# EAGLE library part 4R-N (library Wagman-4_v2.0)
Array Chip Resistor Source: RS Component / Phycomp
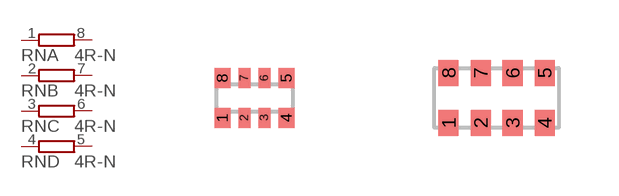
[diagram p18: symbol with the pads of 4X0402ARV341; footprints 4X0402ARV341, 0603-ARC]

Designator prefix RN; gates A=R1NV B=R1NV C=R1NV D=R1NV

## 4R-N0402ARV341 (OC_FARNELL: unknown; OC_NEWARK: unknown)  [4X0402ARV341]
1  A:1  pas
2  B:1  pas
3  C:1  pas
4  D:1  pas
5  D:2  pas
6  C:2  pas
7  B:2  pas
8  A:2  pas

## 4R-N0603-ARC (OC_FARNELL: unknown; OC_NEWARK: unknown)  [0603-ARC]
Pads as for 4X0402ARV341

## 4R-N0603-ARV (OC_FARNELL: unknown; OC_NEWARK: unknown)  [0603-ARV]
Pads as for 4X0402ARV341

## 4R-NCAT16 (OC_FARNELL: unknown; OC_NEWARK: unknown)  [CAT16]
Pads as for 4X0402ARV341

## 4R-NCAY16 (OC_FARNELL: unknown; OC_NEWARK: unknown)  [CAY16]
Pads as for 4X0402ARV341

## 4R-NEXB18V (OC_FARNELL: unknown; OC_NEWARK: unknown)  [EXB18V]
Pads as for 4X0402ARV341

## 4R-NEXB28V (OC_FARNELL: unknown; OC_NEWARK: unknown)  [EXB28V]
Pads as for 4X0402ARV341

## 4R-NEXB38V (OC_FARNELL: unknown; OC_NEWARK: unknown)  [EXB38V]
Pads as for 4X0402ARV341

## 4R-NEXBN8V (OC_FARNELL: unknown; OC_NEWARK: unknown)  [EXBN8V]
Pads as for 4X0402ARV341

## 4R-NEXBS8V (OC_FARNELL: unknown; OC_NEWARK: unknown)  [EXBS8V]
Pads as for 4X0402ARV341

## 4R-NEXBV8V (OC_FARNELL: unknown; OC_NEWARK: unknown)  [EXBV8V]
Pads as for 4X0402ARV341

## 4R-NYC124 (OC_FARNELL: unknown; OC_NEWARK: unknown)  [YC124]
Pads as for 4X0402ARV341

## Footprint 4X0402ARV341 (pad centres in mm)
Array chip resistor size 4 × 0402 Source: http://docs-europe.electrocomponents.com/webdocs/0114/0900766b80114d99.pdf
smd 0.4 x 0.5: 1 -0.8,-0.5; 4 0.8,-0.5; 5 0.8,0.5; 8 -0.8,0.5
smd 0.3 x 0.5: 2 -0.25,-0.5; 3 0.25,-0.5; 6 0.25,0.5; 7 -0.25,0.5

## Footprint 0603-ARC (pad centres in mm)
Chip Resistor Array size 4 × 0603 concave termination - Phycomp Components Source: RS Components
smd 0.5 x 0.65: 1 -1.2,-0.625; 2 -0.4,-0.625; 3 0.4,-0.625; 4 1.2,-0.625; 5 1.2,0.625; 6 0.4,0.625; 7 -0.4,0.625; 8 -1.2,0.625

## Footprint 0603-ARV (pad centres in mm)
Chip Resistor Array size 4 × 0603 convex termination - Phycomp Components Source: RS Components
smd 0.5 x 0.65: 1 -1.2,-0.625; 2 -0.4,-0.625; 3 0.4,-0.625; 4 1.2,-0.625; 5 1.2,0.625; 6 0.4,0.625; 7 -0.4,0.625; 8 -1.2,0.625

## Footprint CAT16 (pad centres in mm)
BOURNS Chip Resistor Array Source: RS Component / BUORNS
smd 0.5 x 0.65: 1 -1.2,-0.675; 2 -0.4,-0.675; 3 0.4,-0.675; 4 1.2,-0.675; 5 1.2,0.675; 6 0.4,0.675; 7 -0.4,0.675; 8 -1.2,0.675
